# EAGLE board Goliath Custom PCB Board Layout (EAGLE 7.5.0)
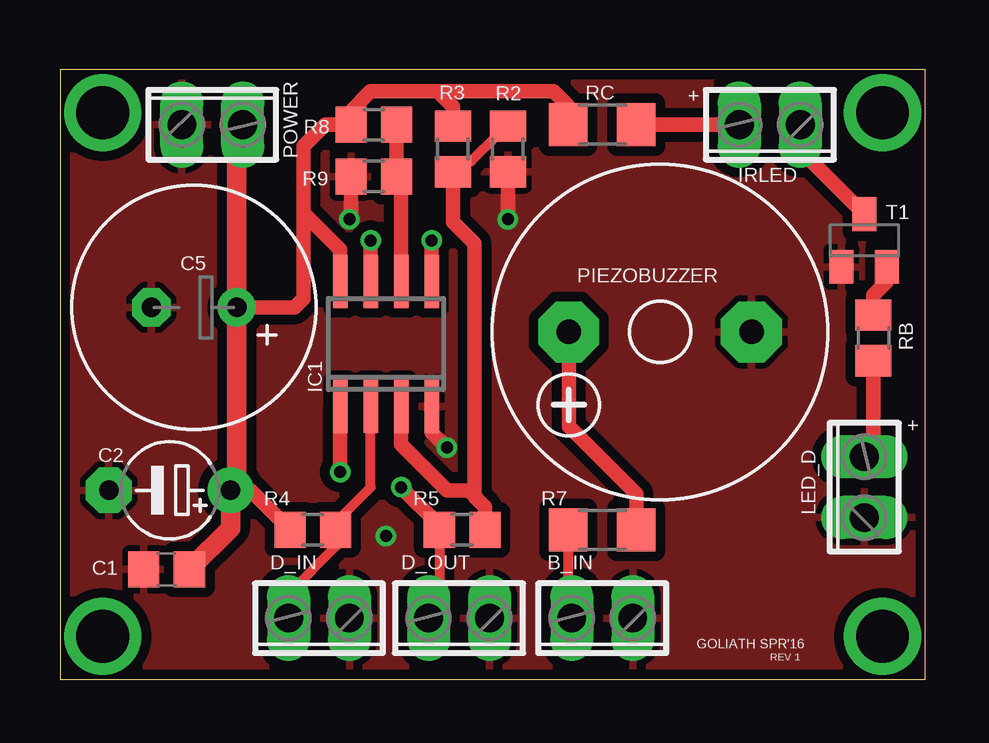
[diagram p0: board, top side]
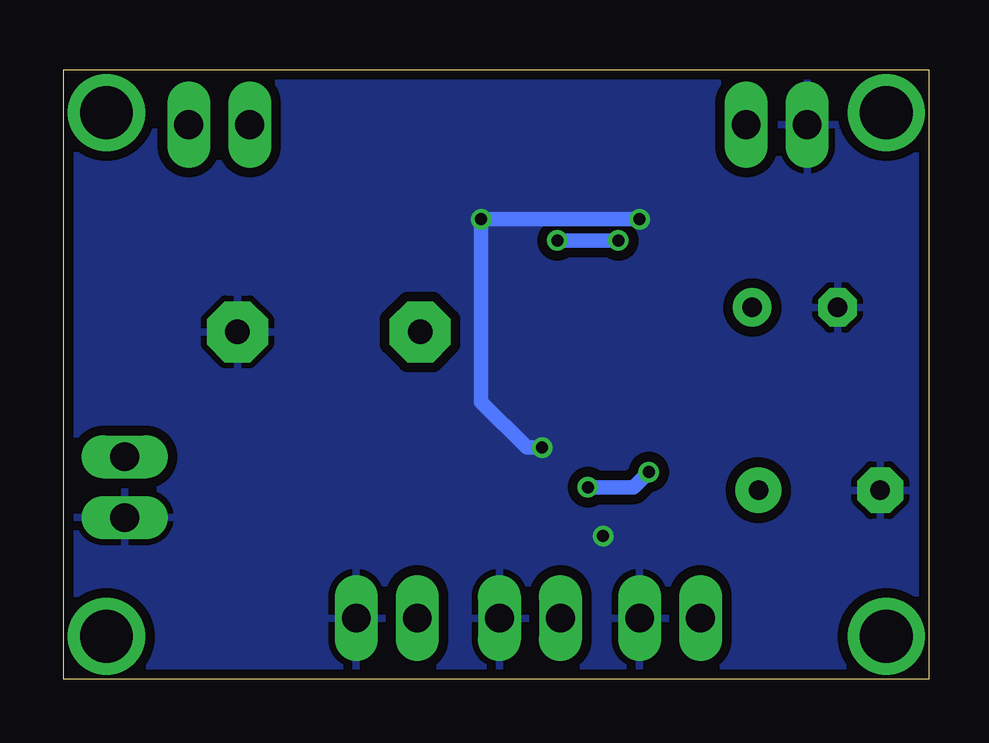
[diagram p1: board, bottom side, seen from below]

Size 36.07 x 25.4 mm. Coordinates in mm from the lower left corner, seen from the top.
Outline: 0,0 36.07,0 36.07,25.4 0,25.4 0,0
Copper layers (1*16): Top 0.0356mm / dielectric 1.5011mm / Bottom 0.0356mm
Design rules "LaenPCBOrder": minimum track width 6mil, minimum drill 13mil, track to track 6mil, track to pad 6mil, pad to pad 6mil, via to via 6mil, smd to smd 6mil, copper to edge 15mil, drill to drill 6mil, minimum pad ring 7mil, minimum via ring 7mil, stop-mask expansion 3mil, vias tented up to drill 0mil, thermal gap 10mil

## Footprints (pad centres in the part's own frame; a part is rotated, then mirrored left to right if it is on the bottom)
2POL254 = drill 1.2 long: 1 -1.27,0; 2 1.27,0
C0805 = smd 1.3 x 1.5: 1 -0.95,0; 2 0.95,0
E5-4 = drill 0.813 pad 1.905: + -2.54,0 | drill 0.813 pad 1.905 octagon: - 2.54,0
E3,5-10 = drill 0.813 pad 1.6: + -1.778,0 | drill 0.813 pad 1.6 octagon: - 1.778,0
SO08 = smd 0.6 x 2.2: 1 -1.905,-2.6; 2 -0.635,-2.6; 3 0.635,-2.6; 4 1.905,-2.6; 5 1.905,2.6; 6 0.635,2.6; 7 -0.635,2.6; 8 -1.905,2.6
F/CM12P = drill 1.016 pad 2.54 octagon: + 3.81,0; - -3.81,0
R0805 = smd 1.3 x 1.5: 1 -0.95,0; 2 0.95,0
R1206 = smd 1.6 x 1.803: 1 -1.422,0; 2 1.422,0
SOT23-EBC = smd 1 x 1.4: B 0.95,-1.1; C 0,1.1; E -0.95,-1.1

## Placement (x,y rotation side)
B_IN  [2POL254]  22.61,2.54 180 top
C1  100nF  [C0805]  4.45,4.57 180 top
C2  10uF  [E5-4]  4.57,7.87 180 top
C5  470uF 10V  [E3,5-10]  5.59,15.49 180 top
D_IN  phototransistor  [2POL254]  10.79,2.54 180 top
D_OUT  output  [2POL254]  16.64,2.54 180 top
IC1  LM358D  [SO08]  13.59,13.97 0 top
IRLED  IRLED  [2POL254]  29.59,23.11 180 top
LED_D  input  [2POL254]  33.53,8 90 top
PIEZOBUZZER  F/CM12P  [F/CM12P]  25.02,14.48 180 top
POWER  5V input  [2POL254]  6.35,23.11 0 top
R2  50k ohm  [R0805]  18.67,22.1 270 top
R3  50k ohm  [R0805]  16.38,22.1 90 top
R4  100k ohm  [R0805]  10.54,6.22 0 top
R5  150k ohm  [R0805]  16.76,6.22 180 top
R7  220 ohm  [R1206]  22.61,6.22 180 top
R8  100K  [R0805]  13.08,23.11 180 top
R9  100k  [R0805]  13.08,20.95 0 top
RB  8.6k ohm  [R0805]  33.91,14.22 90 top
RC  110 ohm  [R1206]  22.61,23.11 180 top
T1  2n2222  [SOT23-EBC]  33.53,18.29 0 top

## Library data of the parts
B_IN D_IN D_OUT IRLED LED_D POWER = con-phoenix-254; OC_FARNELL: unknown; OC_NEWARK: unknown
C1 C2 C5 R2-R5 R7-R9 RB RC = rcl
IC1 = linear
PIEZOBUZZER = buzzer; OC_FARNELL: unknown; OC_NEWARK: unknown
T1 = transistor

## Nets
+5V: C1.1 C2.+ C5.+ IC1.8 POWER.2 R3.2 R4.1 R8.2 RC.2
GND: B_IN.1 C1.2 C2.- C5.- D_IN.1 D_OUT.1 IC1.4 LED_D.1 PIEZOBUZZER.- POWER.1 R2.2 R9.1 T1.E
N$1: D_OUT.2 IC1.1 R5.2
N$2: PIEZOBUZZER.+ R7.1
N$3: D_IN.2 IC1.2 R4.2
N$5: B_IN.2 R7.2
N$6: IC1.3 R2.1 R3.1 R5.1
N$7: IRLED.2 RC.1
N$10: IRLED.1 T1.C
N$11: RB.2 T1.B
N$12: LED_D.2 RB.1
N$14: IC1.5 IC1.7
N$15: IC1.6 R8.1 R9.2

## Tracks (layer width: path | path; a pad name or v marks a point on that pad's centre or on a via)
+5V
  Top 0.61: C2.+ 7.94,7.87 R4.1 | C5.+ 9.78,15.49 10.16,15.88 10.16,19.43 | 10.16,19.43 10.16,22.23 11.05,23.11 R8.2 12.13,23.69 12.95,24.51 15.75,24.51 | IC1.8 11.68,17.91 10.16,19.43 | 15.75,24.51 16.38,23.88 R3.2 | RC.2 21.18,23.9 20.57,24.51 15.75,24.51
  Top 0.813: C1.1 7.11,6.29 C2.+ 7.37,8.13 C5.+ 7.37,22.86 POWER.2
GND  (via drill 0.5)
  Top 0.61: R9.1 12.13,19.49 v12.06,19.18 | v18.67,19.18 R2.2 | IC1.4 15.49,10.29 v16.13,9.65
  Bottom 0.61: v12.06,19.18 v18.67,19.18 18.67,11.56 16.76,9.65 v16.13,9.65
  other vias: 13.59,5.97
  pour Bottom (isolate 0.406): 0,25.4 36.2,25.4 36.2,0 0,0
  pour Top (isolate 0.406): 0,25.4 36.2,25.4 36.2,0 0,0
N$1  (via drill 0.5, 0.5 pad 0.25)
  Top 0.406: D_OUT.2 15.81,2.99 R5.2 15.81,6.41
  Top 0.61: 15.81,6.41 v14.22,8 | v11.68,8.64 IC1.1
  Bottom 0.61: v14.22,8 12.32,8 v11.68,8.64
N$2
  Top 0.61: R7.1 24.03,7.72 21.21,10.54 PIEZOBUZZER.+
N$3
  Top 0.406: IC1.2 12.95,8 11.49,6.54 R4.2 11.56,6.16 11.56,5.59 9.53,3.56 D_IN.2
N$4  (via drill 2.2)
  other vias: 1.78,23.62
N$5
  Top 0.406: R7.2 21.18,2.69 B_IN.2
N$6
  Top 0.406: R5.1 17.71,6.29 | 18.28,23.05 18.28,22.73 17.14,21.59 16.82,21.59 R3.1
  Top 0.61: IC1.3 14.22,9.78 16.13,7.87 17.02,7.87 17.27,7.62 | R3.1 16.38,19.05 17.27,18.16 17.27,7.62 | R2.1 18.28,23.05 | 17.71,6.29 17.71,7.18 17.27,7.62
N$7
  Top 0.61: RC.1 IRLED.2
N$8  (via drill 2.2)
  other vias: 1.78,1.78
N$9  (via drill 2.2 pad 0.25)
  other vias: 34.29,23.62
N$10
  Top 0.61: IRLED.1 30.86,22.05 T1.C
N$11
  Top 0.61: T1.B 34.48,16.57 33.91,16 RB.2
N$12
  Top 0.61: RB.1 33.91,9.65 LED_D.2
N$13  (via drill 2.2)
  other vias: 34.29,1.78
N$14  (via drill 0.5 pad 0.3)
  Top 0.61: IC1.7 v12.95,18.29 | v15.49,18.29 IC1.5
  Bottom 0.61: v12.95,18.29 v15.49,18.29
N$15
  Top 0.61: R8.1 R9.2 14.22,20.76 IC1.6

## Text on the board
tPlace: + | + | GOLIATH SPR'16
tNames: REV 1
